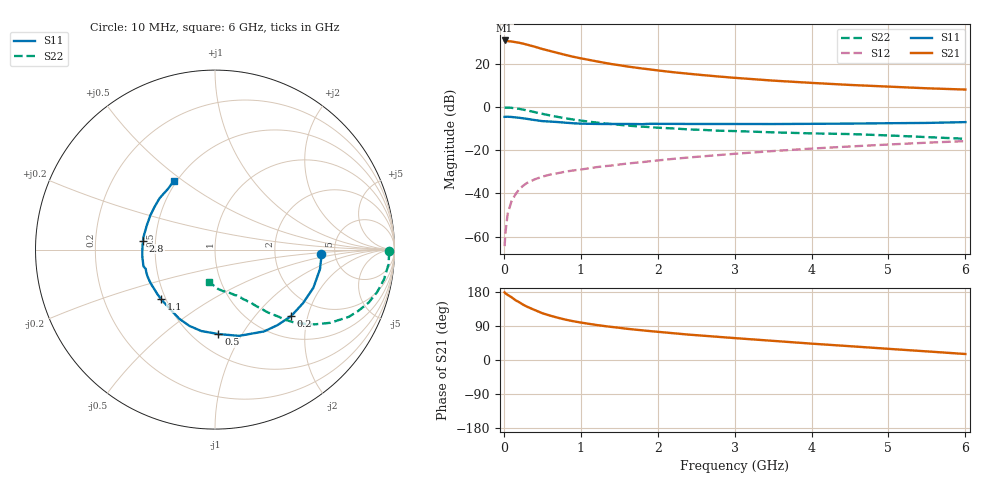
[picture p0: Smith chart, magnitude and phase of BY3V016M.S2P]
! SIEMENS Small Signal Semiconductors
! BFY420
! Si NPN RF SIEGET Grounded Emitter Transistor in MICRO-X
! VCE = 3 V  IC = 16 mA
! Common Emitter S-Parameters:  October  1996
# GHz  S  MA  R  50
!  f  S11  S21  S12  S22
! GHz  MAG  ANG  MAG  ANG  MAG  ANG  MAG  ANG
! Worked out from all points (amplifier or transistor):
!   36 points, 10 MHz to 6 GHz, reference 50 ohm
!   highest |S21| = 30.8 dB at 10 MHz (marker M1)
!   |S21| within 3 dB of that: start of sweep to 410.7 MHz
!   unconditionally stable (mu >= 1): 2.165 GHz to end of sweep
!   at 250 MHz: K = 0.27, MSG = 32.9 dB, |S12| = -36.5 dB
!   at 1.4 GHz: K = 0.86, MSG = 23.5 dB, |S12| = -27.1 dB
!   at 6 GHz: K = 1.07, MAG = 10.3 dB, |S12| = -15.8 dB
!   S11 on the Smith chart (normalised r, x): 10 MHz: 3.88, -0.30; 200 MHz: 1.46, -1.58; 500 MHz: 0.66, -0.79; 1.1 GHz: 0.47, -0.31; 2.8 GHz: 0.43, +0.05; 6 GHz: 0.48, +0.46
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0.01  0.5919 -2.4  34.69 178.5  0.0006 84.7  0.9696 -0.6
0.02  0.5938 -4.2  34.38 175.9  0.0012 84.1  0.97 -1.5
0.05  0.595 -10.5  33.45 171.8  0.0034 88.2  0.9706 -4.8
0.1  0.5879 -21.2  32.88 165.6  0.0066 81.0  0.9561 -10.0
0.15  0.574 -31.4  31.72 158.0  0.0094 74.2  0.9338 -14.7
0.2  0.5633 -41.1  30.68 152.4  0.0125 72.9  0.9059 -19.0
0.25  0.5462 -50.4  29.29 146.1  0.015 68.5  0.8688 -23.1
0.3  0.5315 -59.1  27.79 140.8  0.0174 67.3  0.8353 -26.6
0.4  0.499 -74.4  24.88 132.0  0.0211 62.7  0.7612 -32.4
0.5  0.4708 -87.7  22.03 123.5  0.0244 60.6  0.6951 -36.8
0.6  0.4601 -99.5  19.82 117.2  0.0272 58.0  0.6377 -40.3
0.8  0.4337 -117.2  16.05 106.6  0.0319 55.4  0.5481 -45.2
0.9  0.42 -124.0  14.57 102.4  0.0339 55.5  0.5134 -46.6
1.1  0.4084 -137.4  12.38 95.6  0.0379 55.5  0.4598 -49.8
1.3  0.4036 -146.5  10.61 89.8  0.0425 55.4  0.4184 -51.8
1.6  0.4046 -158.4  8.691 82.4  0.0489 55.5  0.3723 -55.0
2.2  0.4068 -174.4  6.389 70.7  0.0629 54.5  0.3188 -60.2
2.8  0.4043 172.9  5.068 60.9  0.0773 52.3  0.2823 -64.8
3.5  0.4032 160.4  4.078 50.5  0.0955 48.6  0.2589 -70.2
4.5  0.4125 144.7  3.239 36.4  0.1219 41.3  0.2362 -78.8
5.5  0.4277 127.9  2.708 22.7  0.1491 32.7  0.2008 -91.9
6  0.4465 120.7  2.533 15.8  0.1623 28.1  0.1836 -100.5
